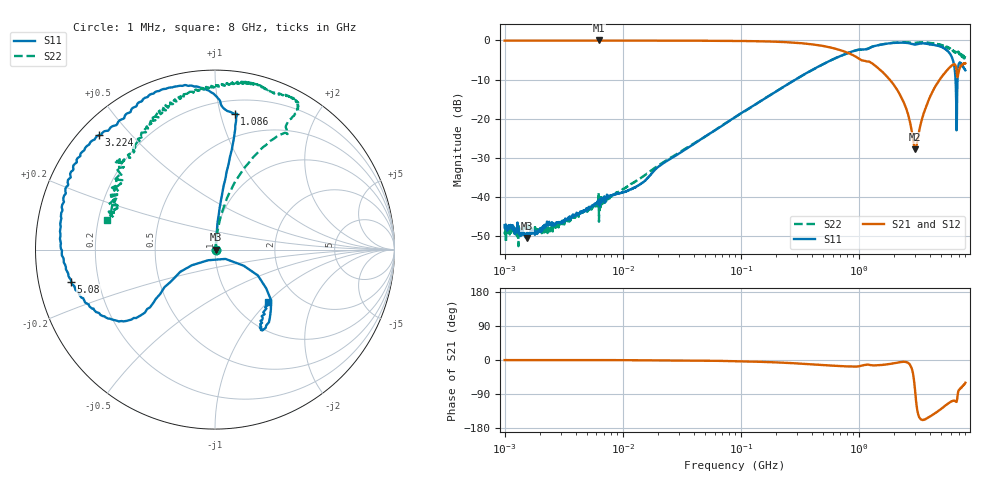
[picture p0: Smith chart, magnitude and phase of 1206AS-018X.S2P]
!s-Parameter Generated by FASTRON Sdn. Bhd.
!FASTRON P/N : 1206AS-018X
!Keysight Technologies: E5071C_MY46733604_B.14.02
!Date: Wed Nov 15 09:44:14 2023
!Version  :Rev00  Wed Nov 15 09:44:14 2023
!Data & Calibration Information:
!Freq  S11:SOLT2(ON)  S21:SOLT2(ON)  S12:SOLT2(ON)  S22:SOLT2(ON)
!PortZ  Port1:50+j0  Port2:50+j0
!When reading reference impedance value at option line is always used.
! Remarks : This data is being provided solely for informational purposes.
# Hz S dB R 50
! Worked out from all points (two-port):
!   1601 points, 1 MHz to 8 GHz, reference 50 ohm
!   highest |S21| = 0.01 dB at 6.301 MHz (marker M1); lowest = -27.9 dB at 3 GHz (marker M2)
!   |S21| within 3 dB of the highest: start of sweep to 783.4 MHz
!   lowest |S11| = -50.5 dB at 1.541 MHz (marker M3), VSWR 1.01, Z = 50.3 - j0.00785 ohm
!   |S11| at or under -10 dB: start of sweep to 290.6 MHz; 6.599 GHz to 6.863 GHz (263.9 MHz wide, 3.92 % of centre)
!   |S22| runs from -52.7 to -0.4 dB; largest |S21 - S12| = 0.0078
!   S11 on the Smith chart (normalised r, x): 1 MHz: 1.01, -0.00; 1.086 GHz: 0.30, +1.11; 3.224 GHz: 0.06, +0.41; 5.08 GHz: 0.10, -0.11; 8 GHz: 1.42, -1.00
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1000000  -47.24 -14.9  -0.03 -0.2  -0.04 -0.1  -48.93 -16.1
1541011  -50.52 -1.5  -0.03 -0.2  -0.03 -0.1  -47.51 -17.0
2198553  -47.15 29.2  -0.03 -0.2  -0.03 -0.2  -48.56 48.1
4479405  -43.69 52.6  -0.04 -0.2  -0.04 -0.2  -44.36 57.9
6301378  -40.84 46.5  0.01 -0.3  -0.06 -0.3  -46.40 52.8
1.345746e7  -37.21 80.5  -0.03 -0.5  -0.05 -0.6  -35.72 70.2
2.00676e7  -32.31 79.0  -0.04 -0.8  -0.05 -0.7  -32.02 78.2
8.994653e7  -19.56 84.4  -0.11 -3.1  -0.12 -3.1  -19.63 82.2
4.006501e8  -7.60 81.6  -0.97 -11.3  -0.98 -11.3  -7.60 72.6
1.086494e9  -2.33 81.8  -5.14 -13.6  -5.15 -13.7  -2.38 58.6
1.7949e9  -0.77 97.2  -9.72 -10.9  -9.74 -11.1  -0.73 59.9
2.457552e9  -0.58 111.8  -16.58 -4.9  -16.62 -5.1  -0.45 63.6
3.000426e9  -1.06 128.1  -27.90 -81.5  -27.92 -81.6  -0.59 71.2
3.223742e9  -0.84 135.4  -23.54 -148.1  -23.58 -148.2  -0.51 74.5
4.216915e9  -1.11 165.2  -13.09 -144.6  -13.08 -144.7  -0.71 88.6
5.080423e9  -1.71 -167.3  -9.11 -126.9  -9.08 -127.1  -1.29 103.2
5.918038e9  -3.39 -144.3  -6.85 -111.9  -6.82 -112.2  -2.08 116.8
6.380696e9  -5.99 -138.8  -6.10 -107.1  -6.07 -107.5  -2.74 128.3
6.65058e9  -12.76 -147.4  -6.73 -109.8  -6.69 -110.3  -2.92 134.3
6.959019e9  -6.83 -46.9  -8.58 -83.1  -8.57 -83.8  -2.83 137.8
7.113238e9  -5.69 -57.1  -7.26 -78.0  -7.25 -78.5  -3.51 141.4
8e9  -7.63 -44.8  -5.84 -60.1  -5.83 -60.6  -4.08 164.9
